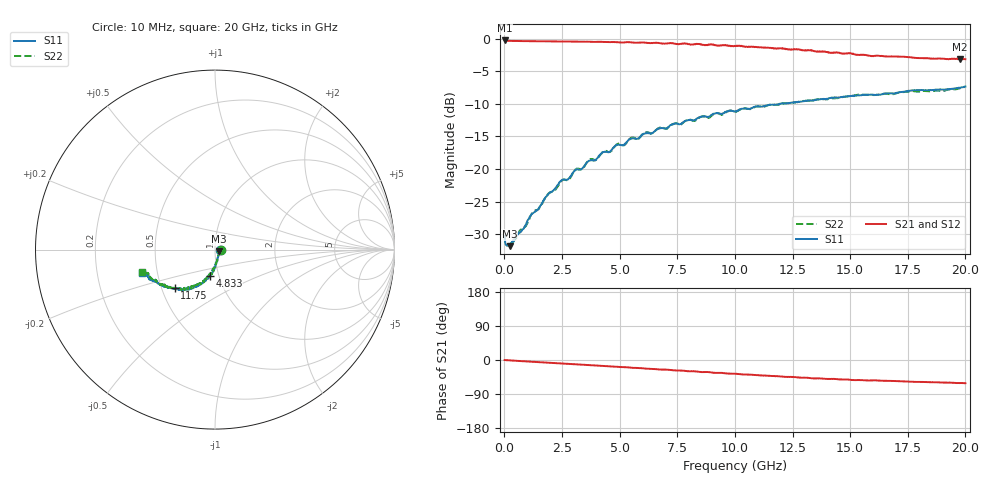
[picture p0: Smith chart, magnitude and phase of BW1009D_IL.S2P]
!  2-Port S-parameters saved by WinCal
! VAR MeasName=S-Parameters (CALIBRATED_DATA) read from VNA (N5244A)
! VAR MeasDate=11/27/2015 2:03:21 PM
! VAR NAME=A150205IL
! VAR FILENAME=A150205IL.S2P
! VAR DATE=11/27/2015 2:03:21 PM
! VAR PHYS_PORTS=1,2
# Hz S DB R 50
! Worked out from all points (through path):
!   801 points, 10 MHz to 20 GHz, reference 50 ohm
!   highest |S21| = -0.29 dB at 10 MHz (marker M1); lowest = -3.2 dB at 19.78 GHz (marker M2)
!   group delay of S21, straight-line fit = 8.86 ps
!   lowest |S11| = -31.8 dB at 234.9 MHz (marker M3), VSWR 1.05, Z = 52.4 - j1.01 ohm
!   |S11| at or under -10 dB: start of sweep to 11.95 GHz
!   |S22| runs from -31.7 to -7.4 dB; largest |S21 - S12| = 0.011
!   S11 on the Smith chart (normalised r, x): 10 MHz: 1.06, -0.01; 4.833 GHz: 0.90, -0.27; 11.75 GHz: 0.58, -0.28; 20 GHz: 0.41, -0.13
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1e7  -30.27 -4.4  -0.29 -0.1  -0.32 -0.2  -30.17 -2.9
1.349375e8  -31.75 -14.4  -0.35 -0.7  -0.34 -0.6  -31.58 -14.5
2.348875e8  -31.82 -21.9  -0.36 -1.0  -0.36 -1.0  -31.56 -20.8
1.884062e9  -23.94 -79.1  -0.44 -7.1  -0.43 -7.1  -23.88 -78.9
2.483762e9  -21.70 -86.9  -0.46 -9.2  -0.46 -9.3  -21.81 -86.7
2.8086e9  -21.41 -88.7  -0.46 -10.4  -0.47 -10.3  -21.56 -88.9
3.10845e9  -20.12 -91.5  -0.48 -11.4  -0.48 -11.5  -20.01 -90.1
3.358325e9  -19.98 -92.7  -0.47 -12.3  -0.48 -12.3  -20.01 -91.2
3.683162e9  -18.74 -94.7  -0.49 -13.6  -0.49 -13.6  -18.59 -94.9
3.983012e9  -18.53 -96.0  -0.51 -14.5  -0.51 -14.5  -18.60 -95.9
4.282862e9  -17.40 -98.6  -0.52 -15.8  -0.53 -15.7  -17.31 -98.6
4.582712e9  -17.30 -99.9  -0.55 -16.7  -0.54 -16.7  -17.38 -99.7
4.832588e9  -16.41 -101.3  -0.54 -17.8  -0.55 -17.9  -16.38 -103.3
5.2074e9  -16.23 -103.1  -0.58 -18.8  -0.59 -19.0  -16.33 -103.7
5.50725e9  -15.33 -106.0  -0.60 -20.4  -0.59 -20.1  -15.18 -105.8
6.681662e9  -13.83 -111.6  -0.66 -24.8  -0.69 -24.6  -13.75 -113.5
1.0005e10  -11.15 -128.7  -1.14 -36.5  -1.16 -36.4  -11.20 -127.8
1.175412e10  -10.13 -136.1  -1.52 -42.8  -1.52 -42.8  -10.16 -135.9
1.335332e10  -9.48 -141.7  -1.85 -47.9  -1.83 -47.8  -9.46 -142.6
1.667666e10  -8.38 -152.6  -2.75 -55.0  -2.77 -54.9  -8.52 -154.1
1.977511e10  -7.53 -161.4  -3.18 -60.8  -3.20 -60.9  -7.62 -162.8
2e10  -7.35 -162.5  -3.17 -61.2  -3.19 -61.0  -7.44 -163.0
